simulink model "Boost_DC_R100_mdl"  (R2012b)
settings: Solver=ode45  StartTime=0.0  StopTime=10.0  RelTol=1e-6  AbsTol=1e-6
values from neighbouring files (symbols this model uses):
  Bg = ones(m,1)    [Boost_DC_M.m]    (also in Boost_DC_R100.m; Boost_Example.m; Boost_DC_Sliding.m)
  C = 200*microF    (= 0.0002)    [Boost_DC_M.m]    (also in Boost_DC_R100.m; Boost_Example.m; Boost_DC_Sliding.m)
  Duty_Cycle = [0.5 0.45 0.48]    [Boost_DC_M.m]    (also in Boost_DC_R100.m = 0.5)
  Im_0 = 0*(1:m)'    [Boost_DC_M.m]    (also in Boost_DC_R100.m; Boost_Example.m = In_Con(jj,1); Boost_DC_Sliding.m = In_Con(jj,1))
  Lm = diag(L1m(1:m))    [Boost_DC_M.m]    (also in Boost_DC_R100.m = eye(m)*L1; Boost_Example.m = eye(m)*L1; Boost_DC_Sliding.m = eye(m)*L1)
  R = 20*Ohm    (= 20)    [Boost_DC_M.m]    (also in Boost_DC_R100.m = 100; Boost_Example.m = 100; Boost_DC_Sliding.m = 100)
  Rm = diag(R1m(1:m))    [Boost_DC_M.m]    (also in Boost_DC_R100.m = eye(m)*R1; Boost_Example.m = eye(m)*R1; Boost_DC_Sliding.m = eye(m)*R1)
  Tc = Ts/50    (= 4e-07)    [Boost_DC_M.m]    (also in Boost_DC_R100.m; Boost_Example.m = 0.0002; Boost_DC_Sliding.m = 2e-05)
  Ts = 0.02*msec    (= 2e-05)    [Boost_DC_M.m]    (also in Boost_DC_R100.m)
  Vc_0 = 0    [Boost_DC_M.m]    (also in Boost_DC_R100.m; Boost_Example.m = In_Con(jj,2); Boost_DC_Sliding.m = In_Con(jj,2))
  Vg = 100*Volt    (= 100)    [Boost_DC_M.m]    (also in Boost_DC_R100.m; Boost_Example.m; Boost_DC_Sliding.m)
undefined symbols (not defined in the file or in its folder): sgn
libraries: simulink x1

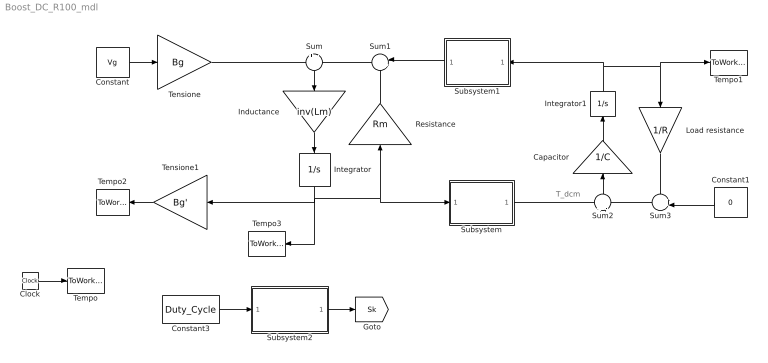
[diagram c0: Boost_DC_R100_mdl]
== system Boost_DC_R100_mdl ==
  note: T_dcm
  Capacitor : Gain  Gain=1/C
  Clock : Clock
  Constant : Constant  Value=Vg
  Constant1 : Constant  Value=0
  Constant3 : Constant  Value=Duty_Cycle
  Inductance : Gain  Gain=inv(Lm)  Multiplication=Matrix(K*u) (u vector)
  Integrator : Integrator  InitialCondition=Im_0  LimitOutput=on  LowerSaturationLimit=0
  Integrator1 : Integrator  InitialCondition=Vc_0
  Load resistance : Gain  Gain=1/R
  Resistance : Gain  Gain=Rm  Multiplication=Matrix(K*u) (u vector)
  Subsystem : Subsystem
  Subsystem1 : Subsystem
  Subsystem2 : Subsystem
  Sum : Sum  Inputs=+|-
  Sum1 : Sum  Inputs=|++
  Sum2 : Sum  Inputs=+|-
  Sum3 : Sum  Inputs=++|
  Tempo : ToWorkspace  VariableName=t  SampleTime=Tc
  Tempo1 : ToWorkspace  VariableName=Vc  SampleTime=Tc
  Tempo2 : ToWorkspace  VariableName=Idc  SampleTime=Tc
  Tempo3 : ToWorkspace  VariableName=Im  SampleTime=Tc
  Tensione : Gain  Gain=Bg  Multiplication=Matrix(K*u) (u vector)
  Tensione1 : Gain  Gain=Bg'  Multiplication=Matrix(K*u) (u vector)
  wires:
  Clock/1 -> Tempo/1
  Sum/1 -> Inductance/1
  Inductance/1 -> Integrator/1
  Integrator/1 -> Resistance/1, Subsystem/1(In1), Tempo3/1, Tensione1/1
  Sum1/1 -> Sum/2
  Resistance/1 -> Sum1/2
  Subsystem/1(Out1) -> Sum2/1
  Sum2/1 -> Capacitor/1
  Capacitor/1 -> Integrator1/1
  Integrator1/1 -> Load resistance/1, Tempo1/1, Subsystem1/1(In1)
  Load resistance/1 -> Sum3/1
  Sum3/1 -> Sum2/2
  Constant1/1 -> Sum3/2
  Subsystem1/1(Out1) -> Sum1/1
  Constant/1 -> Tensione/1
  Tensione/1 -> Sum/1
  Tensione1/1 -> Tempo2/1
  Subsystem2/1(Out1) -> [Sk]
  Constant3/1 -> Subsystem2/1(In1)

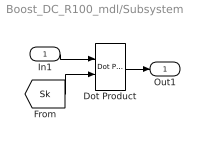
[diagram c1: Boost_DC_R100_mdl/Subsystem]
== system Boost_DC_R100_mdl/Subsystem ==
  In1 : Inport
  Dot Product : simulink/Math Operations/Dot Product  InputSameDT=on  OutDataType=sfix(16)  OutScaling=2^-10  DoSatur=off
  Out1 : Outport
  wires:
  [Sk] -> Dot Product/2
  In1/1 -> Dot Product/1
  Dot Product/1 -> Out1/1

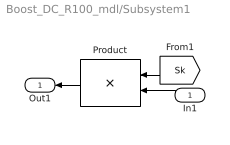
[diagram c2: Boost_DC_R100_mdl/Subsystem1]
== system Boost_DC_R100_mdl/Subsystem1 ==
  In1 : Inport
  Product : Product  Multiplication=Matrix(*)
  Out1 : Outport
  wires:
  [Sk] -> Product/1
  In1/1 -> Product/2
  Product/1 -> Out1/1

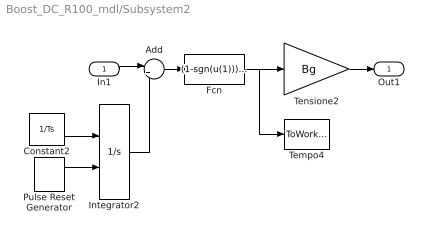
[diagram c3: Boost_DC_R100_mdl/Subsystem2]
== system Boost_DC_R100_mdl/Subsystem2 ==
  In1 : Inport
  Add : Sum  Inputs=|+-
  Constant2 : Constant  Value=1/Ts
  Fcn : Fcn  Expr=(1-sgn(u(1)))/2
  Integrator2 : Integrator  ExternalReset=rising
  Pulse Reset Generator : DiscretePulseGenerator  PulseType=Time based  Period=Ts  PulseWidth=50
  Tempo4 : ToWorkspace  VariableName=S1  SampleTime=Tc
  Tensione2 : Gain  Gain=Bg  Multiplication=Matrix(K*u) (u vector)
  Out1 : Outport
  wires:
  Pulse Reset Generator/1 -> Integrator2/2
  Constant2/1 -> Integrator2/1
  Integrator2/1 -> Add/2
  Add/1 -> Fcn/1
  Fcn/1 -> Tensione2/1, Tempo4/1
  In1/1 -> Add/1
  Tensione2/1 -> Out1/1
